(* Logix 5000 AddOnInstructionDefinition export Banner_R90C_R95C_R130C_Param_v4; software revision 33.00; part 3 of 3 *)
(* tags used below, declared in another part *)
   Hub : Banner_Hub_v4;
   Port_Data : Banner_IOL_Port_v4;
   Port : INT;
   Type : INT;   // 4 = R90C-4B21, 8 = R95C-8B21, 22 = R95-8B22
   Control : DINT;
   Command_Being_Processed : BOOL;
   Update_Archive : BOOL;
   Index_Write_Inprocess : INT;
   Inprocess_Index : DINT;
   Index5 : SINT;
(* Banner_R90C_R95C_R130C_Param_v4, continued *)

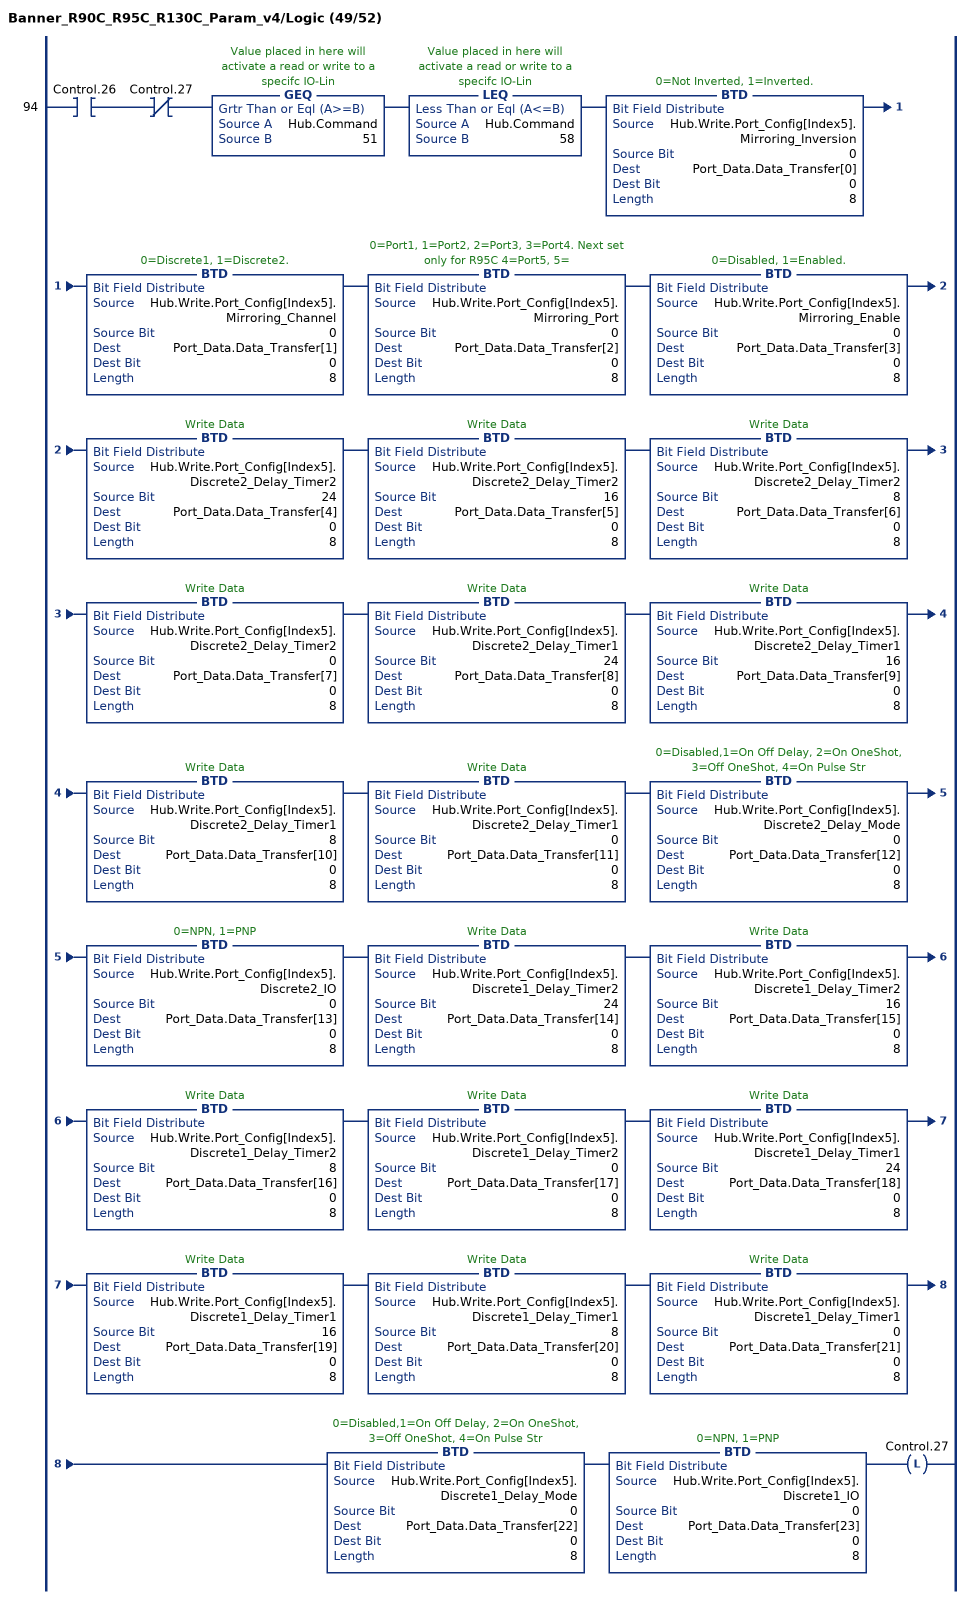
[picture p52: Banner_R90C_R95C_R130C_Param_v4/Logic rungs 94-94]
   94: XIC(Control.26)XIO(Control.27)GEQ(Hub.Command,51)LEQ(Hub.Command,58)BTD(Hub.Write.Port_Config[Index5].Mirroring_Inversion,0,Port_Data.Data_Transfer[0],0,8)BTD(Hub.Write.Port_Config[Index5].Mirroring_Channel,0,Port_Data.Data_Transfer[1],0,8)BTD(Hub.Write.Port_Config[Index5].Mirroring_Port,0,Port_Data.Data_Transfer[2],0,8)BTD(Hub.Write.Port_Config[Index5].Mirroring_Enable,0,Port_Data.Data_Transfer[3],0,8)BTD(Hub.Write.Port_Config[Index5].Discrete2_Delay_Timer2,24,Port_Data.Data_Transfer[4],0,8)BTD(Hub.Write.Port_Config[Index5].Discrete2_Delay_Timer2,16,Port_Data.Data_Transfer[5],0,8)BTD(Hub.Write.Port_Config[Index5].Discrete2_Delay_Timer2,8,Port_Data.Data_Transfer[6],0,8)BTD(Hub.Write.Port_Config[Index5].Discrete2_Delay_Timer2,0,Port_Data.Data_Transfer[7],0,8)BTD(Hub.Write.Port_Config[Index5].Discrete2_Delay_Timer1,24,Port_Data.Data_Transfer[8],0,8)BTD(Hub.Write.Port_Config[Index5].Discrete2_Delay_Timer1,16,Port_Data.Data_Transfer[9],0,8)BTD(Hub.Write.Port_Config[Index5].Discrete2_Delay_Timer1,8,Port_Data.Data_Transfer[10],0,8)BTD(Hub.Write.Port_Config[Index5].Discrete2_Delay_Timer1,0,Port_Data.Data_Transfer[11],0,8)BTD(Hub.Write.Port_Config[Index5].Discrete2_Delay_Mode,0,Port_Data.Data_Transfer[12],0,8)BTD(Hub.Write.Port_Config[Index5].Discrete2_IO,0,Port_Data.Data_Transfer[13],0,8)BTD(Hub.Write.Port_Config[Index5].Discrete1_Delay_Timer2,24,Port_Data.Data_Transfer[14],0,8)BTD(Hub.Write.Port_Config[Index5].Discrete1_Delay_Timer2,16,Port_Data.Data_Transfer[15],0,8)BTD(Hub.Write.Port_Config[Index5].Discrete1_Delay_Timer2,8,Port_Data.Data_Transfer[16],0,8)BTD(Hub.Write.Port_Config[Index5].Discrete1_Delay_Timer2,0,Port_Data.Data_Transfer[17],0,8)BTD(Hub.Write.Port_Config[Index5].Discrete1_Delay_Timer1,24,Port_Data.Data_Transfer[18],0,8)BTD(Hub.Write.Port_Config[Index5].Discrete1_Delay_Timer1,16,Port_Data.Data_Transfer[19],0,8)BTD(Hub.Write.Port_Config[Index5].Discrete1_Delay_Timer1,8,Port_Data.Data_Transfer[20],0,8)BTD(Hub.Write.Port_Config[Index5].Discrete1_Delay_Timer1,0,Port_Data.Data_Transfer[21],0,8)BTD(Hub.Write.Port_Config[Index5].Discrete1_Delay_Mode,0,Port_Data.Data_Transfer[22],0,8)BTD(Hub.Write.Port_Config[Index5].Discrete1_IO,0,Port_Data.Data_Transfer[23],0,8)OTL(Control.27);
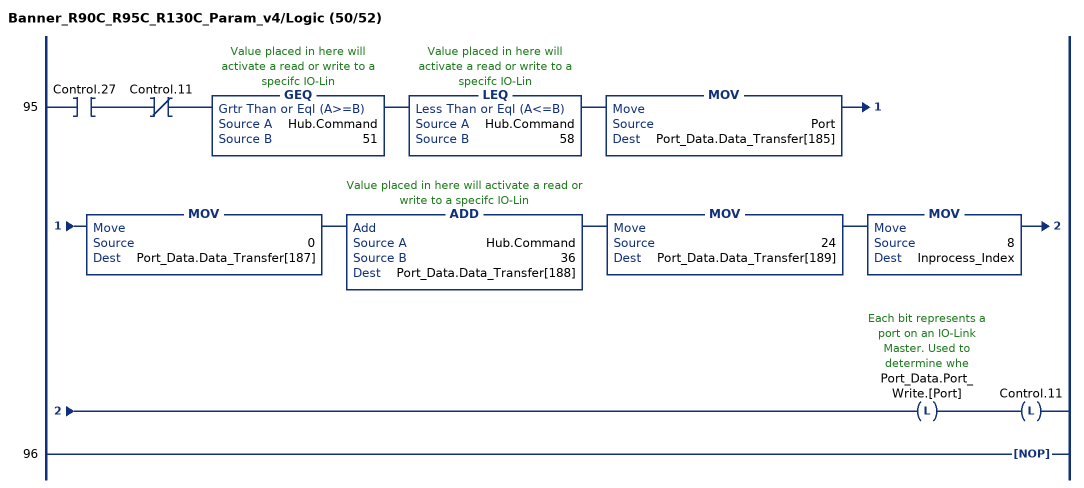
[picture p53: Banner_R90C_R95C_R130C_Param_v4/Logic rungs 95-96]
   95: XIC(Control.27)XIO(Control.11)GEQ(Hub.Command,51)LEQ(Hub.Command,58)MOV(Port,Port_Data.Data_Transfer[185])MOV(0,Port_Data.Data_Transfer[187])ADD(Hub.Command,36,Port_Data.Data_Transfer[188])MOV(24,Port_Data.Data_Transfer[189])MOV(8,Inprocess_Index)OTL(Port_Data.Port_Write.[Port])OTL(Control.11);
   96: NOP();
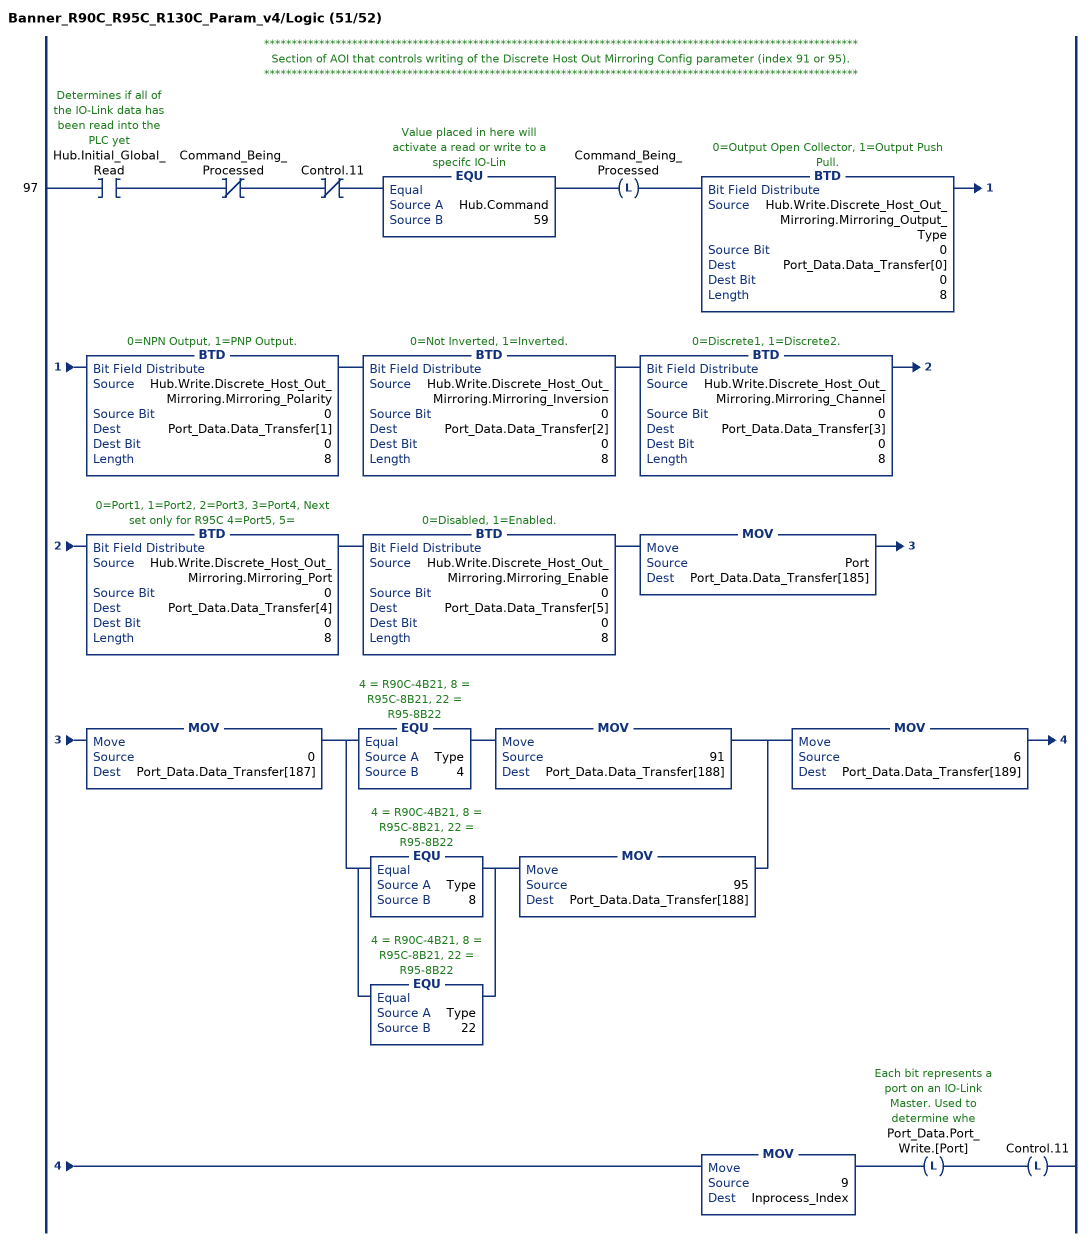
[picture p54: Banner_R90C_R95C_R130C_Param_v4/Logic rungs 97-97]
   // ************************************************************************************************************
   // Section of AOI that controls writing of the Discrete Host Out Mirroring Config parameter (index 91 or 95).
   // ************************************************************************************************************
   97: XIC(Hub.Initial_Global_Read)XIO(Command_Being_Processed)XIO(Control.11)EQU(Hub.Command,59)OTL(Command_Being_Processed)BTD(Hub.Write.Discrete_Host_Out_Mirroring.Mirroring_Output_Type,0,Port_Data.Data_Transfer[0],0,8)BTD(Hub.Write.Discrete_Host_Out_Mirroring.Mirroring_Polarity,0,Port_Data.Data_Transfer[1],0,8)BTD(Hub.Write.Discrete_Host_Out_Mirroring.Mirroring_Inversion,0,Port_Data.Data_Transfer[2],0,8)BTD(Hub.Write.Discrete_Host_Out_Mirroring.Mirroring_Channel,0,Port_Data.Data_Transfer[3],0,8)BTD(Hub.Write.Discrete_Host_Out_Mirroring.Mirroring_Port,0,Port_Data.Data_Transfer[4],0,8)BTD(Hub.Write.Discrete_Host_Out_Mirroring.Mirroring_Enable,0,Port_Data.Data_Transfer[5],0,8)MOV(Port,Port_Data.Data_Transfer[185])MOV(0,Port_Data.Data_Transfer[187])[EQU(Type,4) MOV(91,Port_Data.Data_Transfer[188]) ,[EQU(Type,8) ,EQU(Type,22) ] MOV(95,Port_Data.Data_Transfer[188]) ]MOV(6,Port_Data.Data_Transfer[189])MOV(9,Inprocess_Index)OTL(Port_Data.Port_Write.[Port])OTL(Control.11);
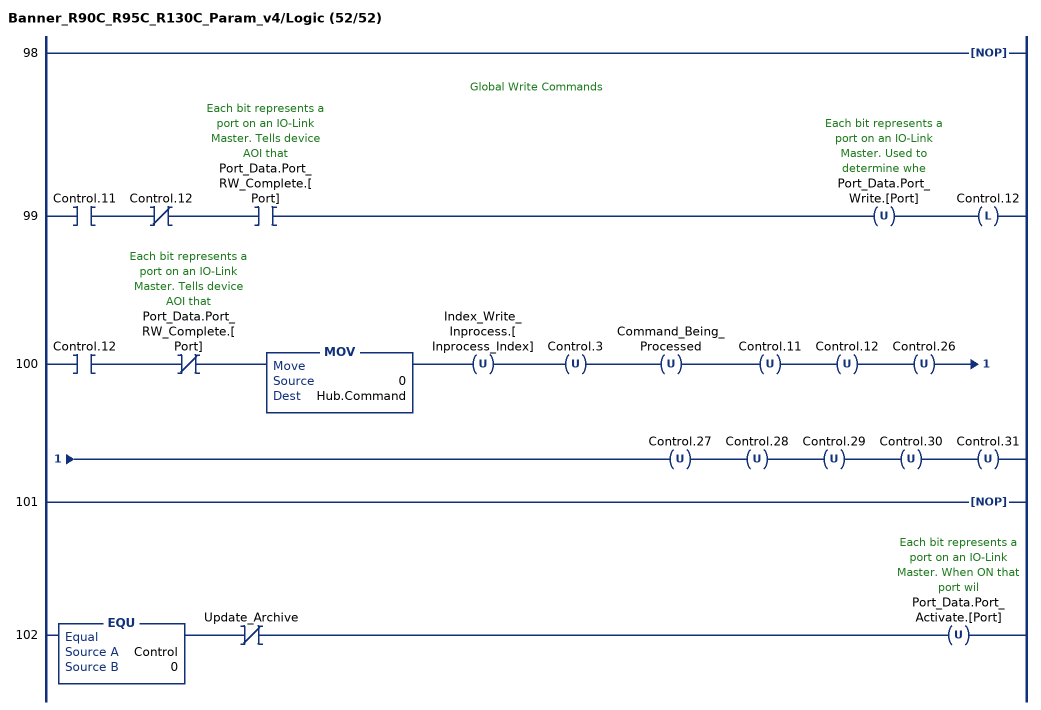
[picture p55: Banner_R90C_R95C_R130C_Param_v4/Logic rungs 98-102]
   98: NOP();
   // Global Write Commands
   99: XIC(Control.11)XIO(Control.12)XIC(Port_Data.Port_RW_Complete.[Port])OTU(Port_Data.Port_Write.[Port])OTL(Control.12);
   100: XIC(Control.12)XIO(Port_Data.Port_RW_Complete.[Port])MOV(0,Hub.Command)OTU(Index_Write_Inprocess.[Inprocess_Index])OTU(Control.3)OTU(Command_Being_Processed)OTU(Control.11)OTU(Control.12)OTU(Control.26)OTU(Control.27)OTU(Control.28)OTU(Control.29)OTU(Control.30)OTU(Control.31);
   101: NOP();
   102: EQU(Control,0)XIO(Update_Archive)OTU(Port_Data.Port_Activate.[Port]);
END_ROUTINE
END_ADD_ON_INSTRUCTION
